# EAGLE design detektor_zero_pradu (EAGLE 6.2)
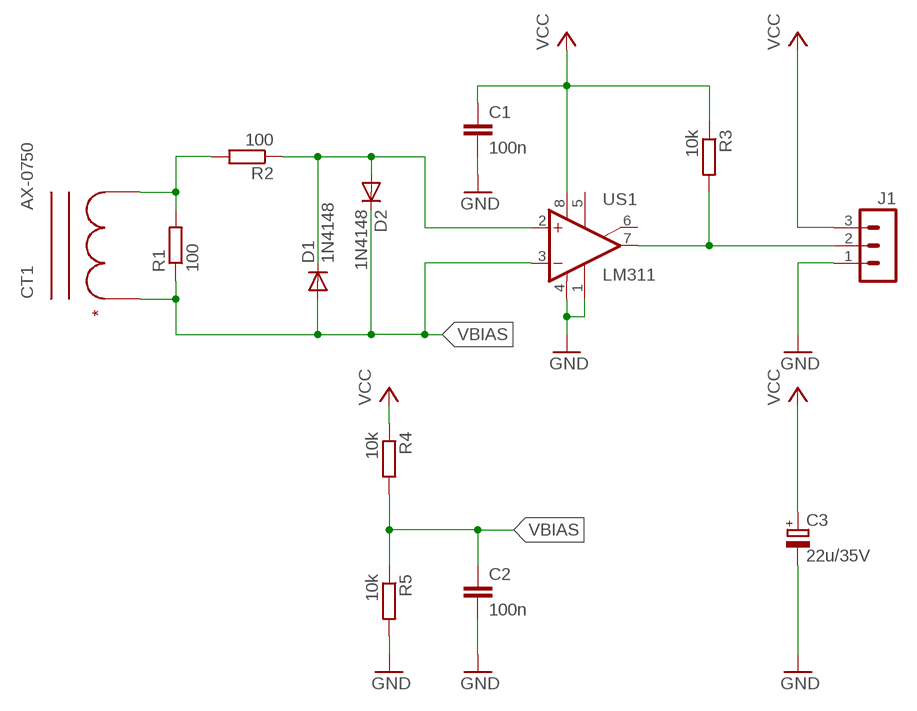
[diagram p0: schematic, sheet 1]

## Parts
C1  100n  C-EUC1206  [C1206]
C2  100n  C-EUC1206  [C1206]
C3  22u/35V  CPOL-EUE2.5-5  [E2,5-5]
CT1  AX-0750  PRZEKLADNIK_I  [PRZEKLADNIK_TALEMA]
D1  1N4148  DIODE-MINIMELF  [MINIMELF]
D2  1N4148  DIODE-MINIMELF  [MINIMELF]
J1  MA03-1  [MA03-1]
R1  100  R-EU_M1206  [M1206]
R2  100  R-EU_M1206  [M1206]
R3  10k  R-EU_M1206  [M1206]
R4  10k  R-EU_M1206  [M1206]
R5  10k  R-EU_M1206  [M1206]
US1  LM311  LM311D  [SO08]

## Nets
GND: C1.2 C2.2 C3.- J1.1 R5.2 US1.1(GND) US1.4(V-)
N$1: D1.C D2.A R2.1 US1.2(+IN)
N$2: J1.2 R3.2 US1.7(OUT)
N$47: CT1.P$2 R1.2 R2.2
VBIAS: C2.1 CT1.P$1 D1.A D2.C R1.1 R4.2 R5.1 US1.3(-IN)
VCC: C1.1 C3.+ J1.3 R3.1 R4.1 US1.8(V+)
Unconnected: US1.5(ON) US1.6(ON/STR)

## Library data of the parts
C1 C2 = rcl:C-EU: CAPACITOR, European symbol
C3 = rcl:CPOL-EU: POLARIZED CAPACITOR, European symbol
CT1 = inne_futrzak:PRZEKLADNIK_I
D1 D2 = diode:DIODE-: DIODE
J1 = con-lstb:MA03-1: PIN HEADER; OC_FARNELL: unknown; OC_NEWARK: unknown
R1-R5 = rcl:R-EU_: RESISTOR, European symbol
US1 = linear:LM311: COMPARATOR

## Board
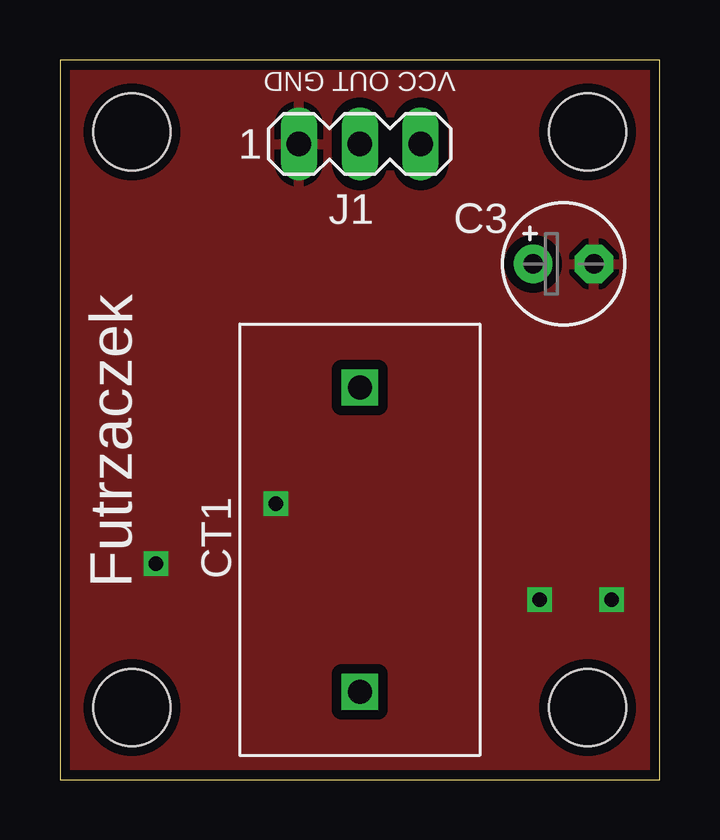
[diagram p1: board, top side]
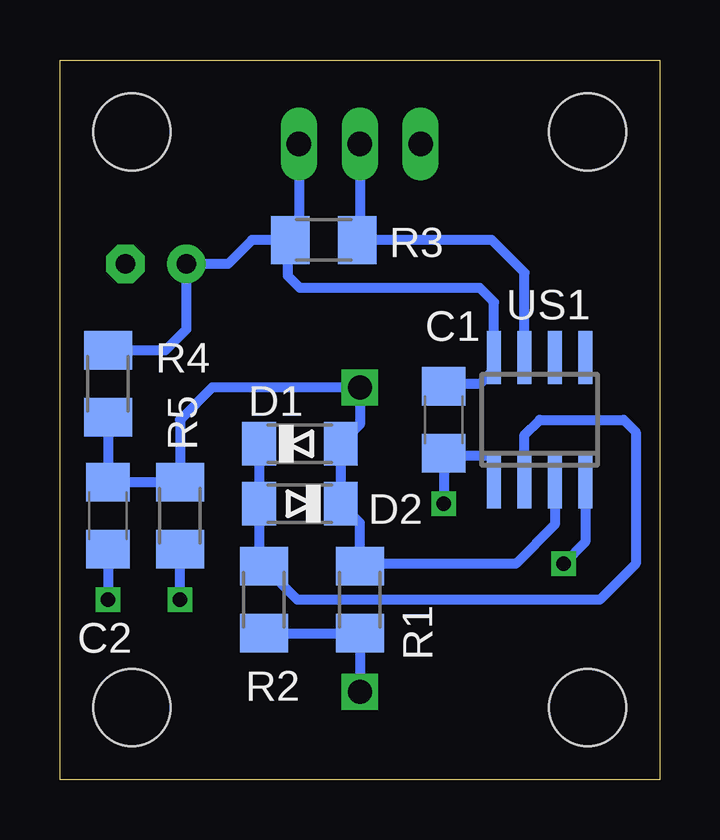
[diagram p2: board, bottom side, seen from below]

Size 25 x 30 mm. Coordinates in mm from the lower left corner, seen from the top.
Outline: 0,0 25,0 25,30 0,30 0,0
Copper layers (1*16): Top 0.035mm / dielectric 1.5mm / Bottom 0.035mm
Design rules: minimum track width 10mil, minimum drill 24mil, track to track 8mil, track to pad 8mil, pad to pad 8mil, via to via 8mil, smd to smd 8mil, copper to edge 10mil, drill to drill 8mil, minimum pad ring 10mil, minimum via ring 8mil, stop-mask expansion 4mil, vias tented up to drill 0mil, thermal gap 10mil
Holes 3.2 mm at 3,3 22,3 3,27 22,27

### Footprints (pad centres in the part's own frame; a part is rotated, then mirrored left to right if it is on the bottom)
C1206 = smd 1.6 x 1.8: 1 -1.4,0; 2 1.4,0
E2,5-5 = drill 0.813 pad 1.6: + -1.27,0 | drill 0.813 pad 1.6 octagon: - 1.27,0
PRZEKLADNIK_TALEMA = drill 1 square: P$1 -6.35,0; P$2 6.35,0
MINIMELF = smd 1.4 x 1.8: A 1.7,0; C -1.7,0
MA03-1 = drill 1.016 long: 1 -2.54,0; 2 0,0; 3 2.54,0
M1206 = smd 1.6 x 2: 1 -1.4,0; 2 1.4,0
SO08 = smd 0.6 x 2.2: 1 -1.905,-2.6; 2 -0.635,-2.6; 3 0.635,-2.6; 4 1.905,-2.6; 5 1.905,2.6; 6 0.635,2.6; 7 -0.635,2.6; 8 -1.905,2.6

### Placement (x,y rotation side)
C1  9,15 270 bottom
C2  23,11 270 bottom
C3  21,21.5 0 top
CT1  12.5,10 270 top
D1  15,14 0 bottom
D2  15,11.5 180 bottom
J1  12.5,26.5 0 top
R1  12.5,7.5 270 bottom
R2  16.5,7.5 270 bottom
R3  14,22.5 0 bottom
R4  23,16.5 270 bottom
R5  20,11 270 bottom
US1  5,15 0 bottom

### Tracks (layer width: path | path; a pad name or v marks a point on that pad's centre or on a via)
GND  (via drill 0.6)
  Bottom 0.406: v9,11.5 C1.2 8.9,13.5 7,13.5 6.91,13.4 US1.1 | C2.2 v23,7.5 | v20,7.5 R5.2 | US1.4 3.1,9.9 v4,9
  pour Top (isolate 0.406): 0,30 25,30 25,0 0,0
N$1
  Bottom 0.406: D1.C D2.A 16.7,9.1 R2.1 15.1,7.5 2.5,7.5 1,9 1,14.5 1.5,15 5,15 5.63,14.37 US1.2
N$2
  Bottom 0.406: US1.7 5.63,21.14 7,22.5 R3.2 12.5,22.6 J1.2
N$47
  Bottom 0.406: CT1.P$2 R1.2 R2.2
VBIAS
  Bottom 0.406: R4.2 C2.1 R5.1 20,15 18.65,16.35 CT1.P$1 12.5,14.8 D1.A D2.C 12.5,10.7 R1.1 12.4,9 6,9 4.37,10.63 US1.3
VCC
  Bottom 0.406: J1.3 15.04,22.86 R3.1 | R3.1 17,22.5 18,21.5 C3.+ 19.73,18.77 20.6,17.9 R4.1 | R3.1 15.5,22.4 15.5,21 15,20.5 7.5,20.5 6.91,19.91 US1.8 6.91,17.09 7.5,16.5 8.9,16.5 C1.1

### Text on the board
tPlace: VCC OUT GND | Futrzaczek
